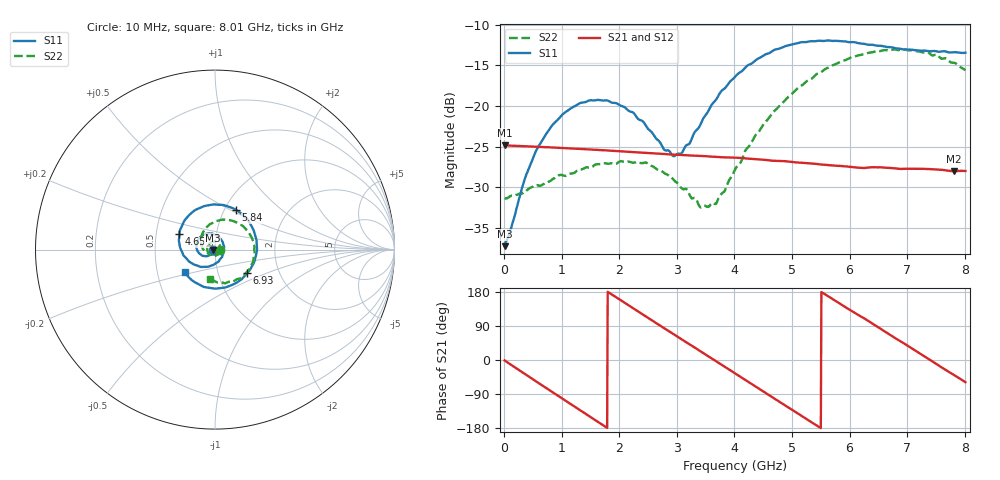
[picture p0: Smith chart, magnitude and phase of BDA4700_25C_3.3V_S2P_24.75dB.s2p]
!Agilent Technologies,E5071B,MY42404982,A.09.10
!Date: Mon Oct 20 18:13:28 2025
!Data & Calibration Information:
!Freq	S11:SOLT2(ON)	S21:SOLT2(ON)	S12:SOLT2(ON)	S22:SOLT2(ON)
# Hz S RI R 50
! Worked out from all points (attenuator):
!   801 points, 10 MHz to 8.01 GHz, reference 50 ohm
!   highest |S21| = -24.82 dB at 10 MHz (marker M1); lowest = -28.0 dB at 7.81 GHz (marker M2)
!   lowest |S11| = -37.2 dB at 10 MHz (marker M3), VSWR 1.03, Z = 48.6 - j0.135 ohm
!   |S11| at or under -10 dB: start of sweep to end of sweep
!   |S22| runs from -32.5 to -13.0 dB; largest |S21 - S12| = 0.00068
!   S11 on the Smith chart (normalised r, x): 10 MHz: 0.97, -0.00; 4.65 GHz: 0.66, +0.12; 5.84 GHz: 1.13, +0.53; 6.93 GHz: 1.38, -0.38; 8.01 GHz: 0.69, -0.18
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1e7  -0.0137 -0.00139  0.0574 -0.00123  0.0574 -0.00129  0.0271 -0.000799
3.7e8  -0.0248 -0.0266  0.0448 -0.0346  0.0447 -0.0346  0.0223 -0.0197
5.8e8  -0.0416 -0.0361  0.0291 -0.048  0.0292 -0.048  0.0144 -0.0292
1e9  -0.0839 -0.0245  -0.0103 -0.0543  -0.0103 -0.0543  -0.0146 -0.0348
1.35e9  -0.1041 0.0132  -0.0388 -0.0381  -0.0389 -0.0381  -0.0365 -0.0183
1.77e9  -0.0837 0.0688  -0.0533 -0.00263  -0.0533 -0.00265  -0.0426 0.0124
2.07e9  -0.0432 0.0892  -0.047 0.0236  -0.047 0.0236  -0.0309 0.0334
2.68e9  0.0413 0.0453  -0.00328 0.0509  -0.00333 0.0509  0.013 0.0383
2.93e9  0.0493 0.00194  0.0176 0.0471  0.0177 0.047  0.025 0.0254
3.06e9  0.0458 -0.0222  0.0275 0.0419  0.027 0.042  0.0278 0.0154
3.43e9  -0.00103 -0.08  0.046 0.0178  0.0461 0.0177  0.02 -0.0129
3.69e9  -0.0558 -0.0954  0.0485 -0.0035  0.0486 -0.00361  0.00146 -0.0253
4.01e9  -0.1309 -0.0749  0.0394 -0.0277  0.0394 -0.0276  -0.0311 -0.0258
4.65e9  -0.1985 0.0856  -0.00608 -0.0457  -0.00591 -0.0458  -0.0787 0.0424
5.35e9  -0.0515 0.2441  -0.0429 -0.0112  -0.0428 -0.0115  -0.0159 0.147
5.84e9  0.1179 0.2202  -0.0363 0.0227  -0.0362 0.0227  0.093 0.1616
6.26e9  0.2161 0.1054  -0.0136 0.0394  -0.013 0.0395  0.1811 0.1032
6.68e9  0.2243 -0.0495  0.0154 0.0387  0.0154 0.0387  0.219 5.1e-05
6.93e9  0.1798 -0.131  0.0291 0.0291  0.0292 0.0289  0.2123 -0.0695
7.37e9  0.0393 -0.2135  0.041 0.00199  0.0409 0.00196  0.138 -0.1618
7.81e9  -0.1186 -0.1777  0.0308 -0.0251  0.0308 -0.0252  0.0173 -0.1834
8.01e9  -0.1698 -0.1275  0.0208 -0.034  0.021 -0.034  -0.0302 -0.1627
